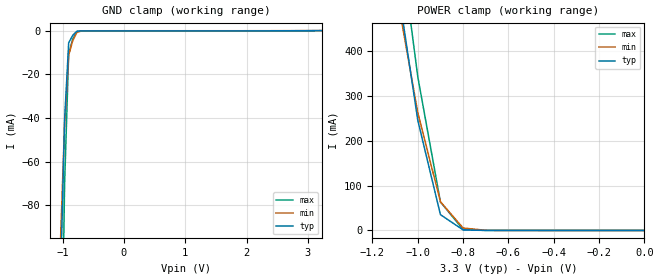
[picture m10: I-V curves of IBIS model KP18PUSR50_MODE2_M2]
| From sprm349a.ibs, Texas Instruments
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|   Model Cell KP18PUSR50_MODE2_M2
[Model]   KP18PUSR50_MODE2_M2
Model_type   Input
Polarity   Non-Inverting
Vinl =  0.8V
Vinh =  2V
C_comp   0.5006264p   0.4551273p   0.5623334p
[Model Spec]
Vinl   0.8V   0.8V   0.8V
Vinh   2V   2V   2V
[Temperature Range]   25   105   0
[Voltage Range]   3.3   3.14   3.47
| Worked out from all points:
|   GND clamp passes 1 mA (typ) near -0.79 V on its own axis
|   POWER clamp passes 1 mA (typ) near -0.78 V on its own axis
[POWER_clamp]
|   voltage   I(typ)   I(min)   I(max)
-3.3V     9.936A     8.589A     10.91A
-1.067V   472.1mA    454mA      602.9mA
-1.033V   359.2mA    358.6mA    473.3mA
-1V       246.3mA    263.1mA    343.6mA
-900mV    35.32mA    64.33mA    63.62mA
-800mV    1.234mA    5.498mA    1.929mA
-700mV    130.3uA    388.1uA    162.6uA
-11.55fV  95.23nA    66.33nA    458.2nA
[GND_clamp]
|   voltage   I(typ)   I(min)   I(max)
-3.3V     -13.46A    -11.58A    -14.63A
-1.033V   -115.5mA   -96.35mA   -194.2mA
-966.7mV  -41.01mA   -42.91mA   -70.35mA
-900mV    -5.577mA   -11.26mA   -10.52mA
-833.3mV  -2.123mA   -4.53mA    -3.817mA
-766.7mV  -314.7uA   -866.3uA   -378.8uA
-700mV    -151.3uA   -264.3uA   -204.6uA
-500mV    -137.1uA   -72.3uA    -191.4uA
3.233V    -8.72uA    8.017uA    -38.34uA
